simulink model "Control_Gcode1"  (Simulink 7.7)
settings: Solver=FixedStepDiscrete  SolverMode=SingleTasking  StartTime=0  StopTime=inf  FixedStep=dt  RelTol=1e-3  SampleTimeConstraint=Specified
InitFcn:
  | % Sampling Times %
  | dt0=0.001; dt1=0.01; samples=10;
undefined symbols (not defined in the file or in its folder): DiscIntNeverNeededParam, Volts
libraries: simulink_extras x4, speedgoatlib_IO311 x3, xpclib x3, simulink x3, speedgoatlib x2

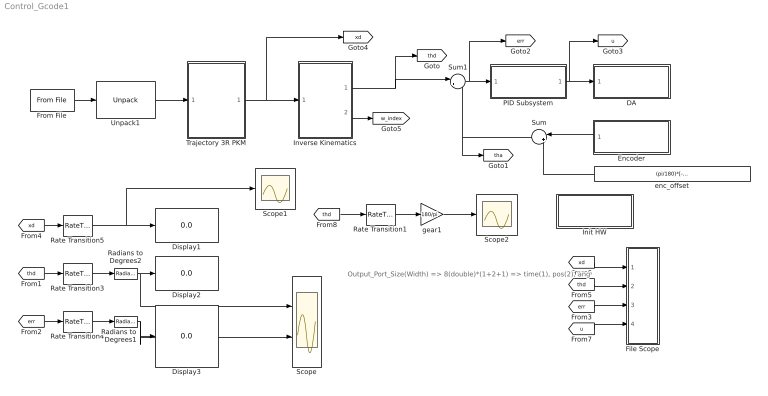
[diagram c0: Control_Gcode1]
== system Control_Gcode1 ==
  note: Output_Port_Size(Width) => 8(double)*(1+2+1) => time(1), pos(2), ang
  DA : Subsystem  TreatAsAtomicUnit=on
  Display1 : Display
  Display2 : Display
  Display3 : Display
  Encoder : Subsystem  TreatAsAtomicUnit=on
  File Scope : Subsystem
  From File : xpclib/Misc./From File  filename='pkm1.dat'  dataSize=32  bufSize=4000  readSize=1024  EOFOption=Hold last output  sampTime=dt0
  Init HW : Subsystem  TreatAsAtomicUnit=on
  Inverse Kinematics : Stateflow chart  TreatAsAtomicUnit=on
  PID Subsystem : Subsystem  TreatAsAtomicUnit=on
  Radians to Degrees1 : simulink_extras/Transformations/Radians to Degrees  SystemSampleTime=-1
  Radians to Degrees2 : simulink_extras/Transformations/Radians to Degrees  SystemSampleTime=-1
  Rate Transition{1,3..5} (4 alike) : RateTransition  OutPortSampleTime=dt1
  Scope : Scope  NumInputPorts=2
  Scope1 : Scope
  Scope2 : Scope
  Sum : Sum  Inputs=|++
  Sum1 : Sum  Inputs=|+-
  Trajectory 3R PKM : Stateflow chart  TreatAsAtomicUnit=on
  Unpack1 : xpclib/UDP/Unpack  dimensions={[4]}  datatypes={'double'}  byteAlign=1
  enc_offset : Constant  Value=(pi/180)*[-144.9004,-24.9004,95.0996]'
  gear1 : Gain  Gain=180/pi
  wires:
  [thd] -> Rate Transition3/1
  [err] -> Rate Transition4/1
  [xd] -> Rate Transition5/1
  Rate Transition5/1 -> Display1/1, Scope1/1
  Rate Transition3/1 -> Radians to Degrees2/1
  Rate Transition4/1 -> Radians to Degrees1/1
  Radians to Degrees2/1 -> Display2/1, Scope/1
  Radians to Degrees1/1 -> Display3/1, Scope/2
  [xd] -> File Scope/1(xd)
  [thd] -> File Scope/2(thd)
  [err] -> File Scope/3(err)
  [u] -> File Scope/4(u)
  From File/1 -> Unpack1/1
  Unpack1/1 -> Trajectory 3R PKM/1(traj)
  Sum1/1 -> PID Subsystem/1(In1), [err]
  PID Subsystem/1(Out1) -> [u], DA/1(In1)
  Encoder/1(Out1) -> Sum/1
  enc_offset/1 -> Sum/2
  Sum/1 -> Sum1/2, [tha]
  Inverse Kinematics/1(thd) -> Sum1/1, [thd]
  Inverse Kinematics/2(w_index) -> [w_index]
  Trajectory 3R PKM/1(xd) -> Inverse Kinematics/1(xd), [xd]
  [thd] -> Rate Transition1/1
  Rate Transition1/1 -> gear1/1
  gear1/1 -> Scope2/1

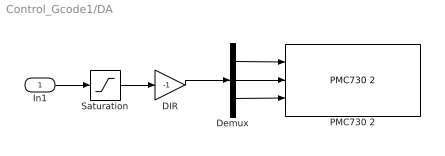
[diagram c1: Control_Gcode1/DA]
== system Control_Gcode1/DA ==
  In1 : Inport
  DIR : Gain  Gain=-1
  Demux : Demux  Outputs=3
  PMC730 2 : speedgoatlib/IO101/PMC730 2  id=1  channel=[1,2,3]  reset=[1,1,1]  initValue=[0,0,0]  ts=dt0  pciSlot=-1
  Saturation : Saturate  UpperLimit=10  LowerLimit=-10
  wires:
  In1/1 -> Saturation/1
  Saturation/1 -> DIR/1
  DIR/1 -> Demux/1
  Demux/1 -> PMC730 2/1
  Demux/2 -> PMC730 2/2
  Demux/3 -> PMC730 2/3

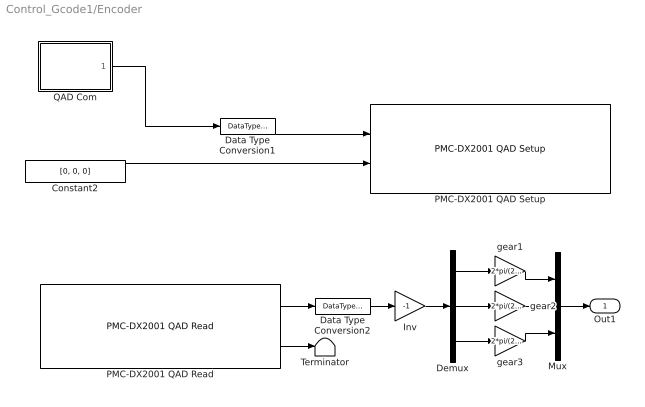
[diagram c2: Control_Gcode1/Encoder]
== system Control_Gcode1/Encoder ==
  Constant2 : Constant  Value=[0, 0, 0]  OutDataTypeStr=Inherit: Inherit via back propagation
  Data Type Conversion1 : DataTypeConversion  OutDataTypeStr=uint8
  Data Type Conversion2 : DataTypeConversion  OutDataTypeStr=double
  Demux : Demux  Outputs=3
  Inv : Gain  Gain=-1
  Mux : Mux  Inputs=3
  PMC-DX2001 QAD Read : speedgoatlib_IO311/PMC-DX2001 QAD Read  id=1  chan=[1, 2, 3]  pciSlot=-1  ts=dt0
  PMC-DX2001 QAD Setup : speedgoatlib_IO311/PMC-DX2001 QAD Setup  id=1  chan=Channel 3 setup  steps1=2000  steps2=2000  steps3=2000  quadrature1=4x  quadrature2=4x  quadrature3=4x  index1=Ignore index input  index2=Ignore index input  index3=Ignore index input  special1=Disabled (cycling counter)  special2=Disabled (cycling counter)  special3=Disabled (cycling counter)  debounce=0  pciSlot=-1  ts=dt0
  QAD Com : Stateflow chart  TreatAsAtomicUnit=on
  Terminator : Terminator
  gear1 : Gain  Gain=2*pi/(23*2000)
  gear2 : Gain  Gain=2*pi/(23*2000)
  gear3 : Gain  Gain=2*pi/(23*2000)
  Out1 : Outport
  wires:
  Constant2/1 -> PMC-DX2001 QAD Setup/2
  PMC-DX2001 QAD Read/2 -> Terminator/1
  PMC-DX2001 QAD Read/1 -> Data Type Conversion2/1
  QAD Com/1(y) -> Data Type Conversion1/1
  Data Type Conversion1/1 -> PMC-DX2001 QAD Setup/1
  Data Type Conversion2/1 -> Inv/1
  Mux/1 -> Out1/1
  Demux/1 -> gear1/1
  gear1/1 -> Mux/1
  Demux/2 -> gear2/1
  gear2/1 -> Mux/2
  Inv/1 -> Demux/1
  Demux/3 -> gear3/1
  gear3/1 -> Mux/3

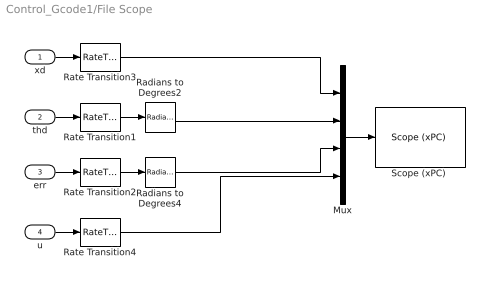
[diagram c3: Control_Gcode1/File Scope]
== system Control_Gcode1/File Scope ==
  xd : Inport
  thd : Inport  Port=2
  err : Inport  Port=3
  u : Inport  Port=4
  Mux : Mux
  Radians to Degrees2 : simulink_extras/Transformations/Radians to Degrees  SystemSampleTime=-1
  Radians to Degrees4 : simulink_extras/Transformations/Radians to Degrees  SystemSampleTime=-1
  Rate Transition{1..4} (4 alike) : RateTransition  OutPortSampleTime=dt1
  "Scope (xPC) " : xpclib/Misc./Scope (xPC)   SystemSampleTime=-1  scopeno=2  scopetype=File  autostart=on  viewmode=Graphical redraw  formatstr='%15.6f'  grid=on  ylimits=[0,0]  nosamples=100  noprepostsamples=0  interleave=1  triggermode=FreeRun  triggersignal=1  triggerlevel=0.0  triggerslope=Either  triggerscope=1  triggersample=0  filename=step3.dat  mode=Lazy  writesize=512  autorestart=on  dynamicfilemode=off  maxwritefilesize=512*1024^2
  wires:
  Radians to Degrees2/1 -> Mux/2
  Radians to Degrees4/1 -> Mux/3
  Rate Transition1/1 -> Radians to Degrees2/1
  Rate Transition2/1 -> Radians to Degrees4/1
  thd/1 -> Rate Transition1/1
  err/1 -> Rate Transition2/1
  Rate Transition3/1 -> Mux/1
  xd/1 -> Rate Transition3/1
  u/1 -> Rate Transition4/1
  Mux/1 -> "Scope (xPC) "/1
  Rate Transition4/1 -> Mux/4

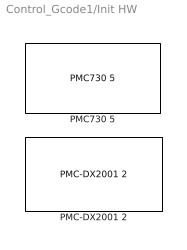
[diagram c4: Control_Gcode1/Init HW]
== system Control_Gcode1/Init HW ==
  PMC-DX2001 2 : speedgoatlib_IO311/PMC-DX2001 2  id=1  fpga1=IO311_3PWM_3CAP_3QAD_INT.fpga  fpga2=PWM_Triangle_DX501.fpga  fpga3=PWM_Triangle_DX501.fpga  fpga4=PWM_Triangle_DX501.fpga  fpga5=PWM_Triangle_DX501.fpga  fpga6=PWM_Triangle_DX501.fpga  fpga7=PWM_Triangle_DX501.fpga  fpga8=PWM_Triangle_DX501.fpga  fpga9=PWM_Triangle_DX501.fpga  fpga10=PWM_Triangle_DX501.fpga  group=Module setup  pciSlot=-1  lowerDirection=[ones(1,5), zeros(1, 7), ones(1, 1), ones(1, 3)]  lowerReset=[1]  lowerValue=[0]  upperDirection=[ones(1, 8), zeros(1, 8)]  upperReset=[1]  upperValue=[0]
  PMC730 5 : speedgoatlib/IO101/PMC730 5  id=1  group=Analog output setup  pciSlot=-1  adStartChannel=1  adNumChannel=1  adCoupling=Single-ended  adRange=-10 .. 10 Volts  adAcqMode=Standard  daChannel=[1,2, 3]  daReset=[1,1, 1]  daInitValue=[0,0,0]  diChannel=[1]  diDebounce=[0]  doChannel=[1]  doReset=[1]  doInitValue=[0]

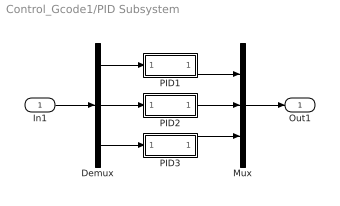
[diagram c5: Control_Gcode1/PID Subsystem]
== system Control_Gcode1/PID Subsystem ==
  In1 : Inport
  Demux : Demux  Outputs=3
  Mux : Mux  Inputs=3
  PID1 : Subsystem
  PID2 : Subsystem
  PID3 : Subsystem
  Out1 : Outport
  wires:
  In1/1 -> Demux/1
  Demux/1 -> PID1/1(In1)
  PID1/1(Out1) -> Mux/1
  Demux/2 -> PID2/1(In1)
  PID2/1(Out1) -> Mux/2
  Mux/1 -> Out1/1
  Demux/3 -> PID3/1(In1)
  PID3/1(Out1) -> Mux/3

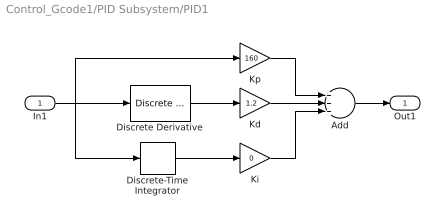
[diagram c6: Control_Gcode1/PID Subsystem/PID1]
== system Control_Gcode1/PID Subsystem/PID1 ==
  In1 : Inport
  Add : Sum  Inputs=+++
  Discrete Derivative : simulink/Discrete/Discrete Derivative  SystemSampleTime=-1  gainval=1.0  ICPrevScaledInput=0.0  OutMin=[]  OutMax=[]  OutDataType=fixdt(1, 16)  OutScaling=2^-10  DoSatur=off
  Discrete-Time Integrator : DiscreteIntegrator  SampleTime=dt0  ICPrevOutput=DiscIntNeverNeededParam  ICPrevScaledInput=DiscIntNeverNeededParam
  Kd : Gain  Gain=1.2
  Ki : Gain  Gain=0
  Kp : Gain  Gain=160
  Out1 : Outport
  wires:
  Discrete-Time Integrator/1 -> Ki/1
  Kp/1 -> Add/1
  Kd/1 -> Add/2
  Ki/1 -> Add/3
  Discrete Derivative/1 -> Kd/1
  Add/1 -> Out1/1
  In1/1 -> Kp/1, Discrete Derivative/1, Discrete-Time Integrator/1

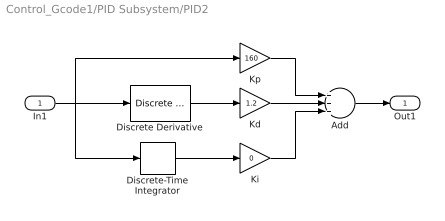
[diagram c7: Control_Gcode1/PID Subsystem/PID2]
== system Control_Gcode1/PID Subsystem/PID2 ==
  In1 : Inport
  Add : Sum  Inputs=+++
  Discrete Derivative : simulink/Discrete/Discrete Derivative  SystemSampleTime=-1  gainval=1.0  ICPrevScaledInput=0.0  OutMin=[]  OutMax=[]  OutDataType=fixdt(1, 16)  OutScaling=2^-10  DoSatur=off
  Discrete-Time Integrator : DiscreteIntegrator  SampleTime=dt0  ICPrevOutput=DiscIntNeverNeededParam  ICPrevScaledInput=DiscIntNeverNeededParam
  Kd : Gain  Gain=1.2
  Ki : Gain  Gain=0
  Kp : Gain  Gain=160
  Out1 : Outport
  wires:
  Discrete-Time Integrator/1 -> Ki/1
  Kp/1 -> Add/1
  Kd/1 -> Add/2
  Ki/1 -> Add/3
  Discrete Derivative/1 -> Kd/1
  Add/1 -> Out1/1
  In1/1 -> Kp/1, Discrete Derivative/1, Discrete-Time Integrator/1

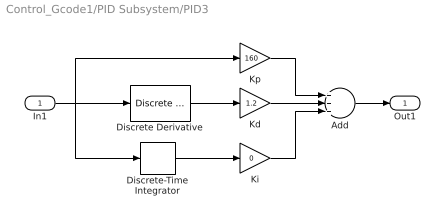
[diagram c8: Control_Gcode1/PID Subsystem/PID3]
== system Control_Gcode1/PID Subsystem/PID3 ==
  In1 : Inport
  Add : Sum  Inputs=+++
  Discrete Derivative : simulink/Discrete/Discrete Derivative  SystemSampleTime=-1  gainval=1.0  ICPrevScaledInput=0.0  OutMin=[]  OutMax=[]  OutDataType=fixdt(1, 16)  OutScaling=2^-10  DoSatur=off
  Discrete-Time Integrator : DiscreteIntegrator  SampleTime=dt0  ICPrevOutput=DiscIntNeverNeededParam  ICPrevScaledInput=DiscIntNeverNeededParam
  Kd : Gain  Gain=1.2
  Ki : Gain  Gain=0
  Kp : Gain  Gain=160
  Out1 : Outport
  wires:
  Discrete-Time Integrator/1 -> Ki/1
  Kp/1 -> Add/1
  Kd/1 -> Add/2
  Ki/1 -> Add/3
  Discrete Derivative/1 -> Kd/1
  Add/1 -> Out1/1
  In1/1 -> Kp/1, Discrete Derivative/1, Discrete-Time Integrator/1

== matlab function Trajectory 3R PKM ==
function xd = fcn(traj)

x0=[0,0,0]';
xd=x0+traj(2:4,1);

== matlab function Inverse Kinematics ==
function [thd,w_index]  = fcn(xd)

persistent index thd_p

% Initializing Variables %
if isempty(index), index=0; end
if isempty(thd_p), thd_p=(pi/180)*[-144.9004,-24.9004,95.0996]'; end

% Kinematic Parameters %
ra=150; rb=35; L1=100; L2=100;

pos=xd(1:2,1); ang=xd(3,1);

w_index=1;  % In workspace %

% Vertex Points %
A=ra*[0,-sqrt(3)/2, +sqrt(3)/2; 1, -1/2, -1/2];
B=rb*[0,-sqrt(3)/2, +sqrt(3)/2; 1, -1/2, -1/2];

th=zeros(3,1);
R=[cos(ang), -sin(ang); sin(ang), cos(ang)];
for i=1:3
    d=pos+R*B(:,i)-A(:,i);
    e1=-2*L1*d(2,1); e2=-2*L1*d(1,1);
    e3=d(1,1)^2+d(2,1)^2+L1^2-L2^2;
    temp=e1^2+e2^2-e3^2;
    if temp>=0
        th(i,1)=2*atan((-e1-sqrt(temp))/(e3-e2));
    else
        th(i,1)=0;
        w_index=-1;
        %disp('Out of Workspace');
    end
end

% Result %
if w_index==1
    thd=[th(1,1), th(2,1), th(3,1)]';
else
    thd=thd_p;
end

% Save the current value %
thd_p=thd;

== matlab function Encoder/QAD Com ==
function y = fcn()

persistent index

if isempty(index), index=0; end

if index==0
    y=[1,1,1];      %  Reset %
else
    y = [0,0,0];
end

index=index+1;
